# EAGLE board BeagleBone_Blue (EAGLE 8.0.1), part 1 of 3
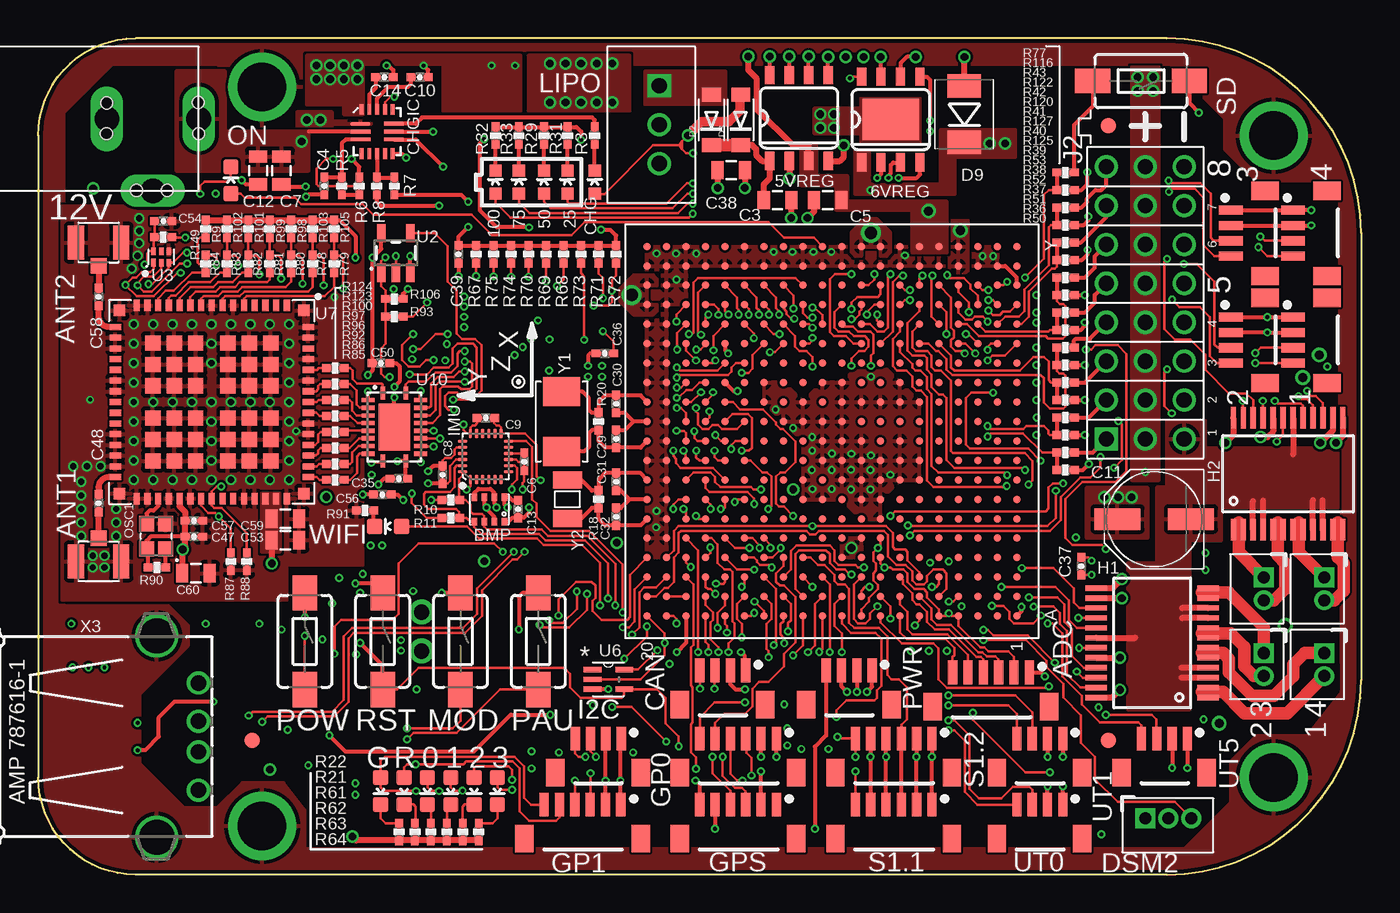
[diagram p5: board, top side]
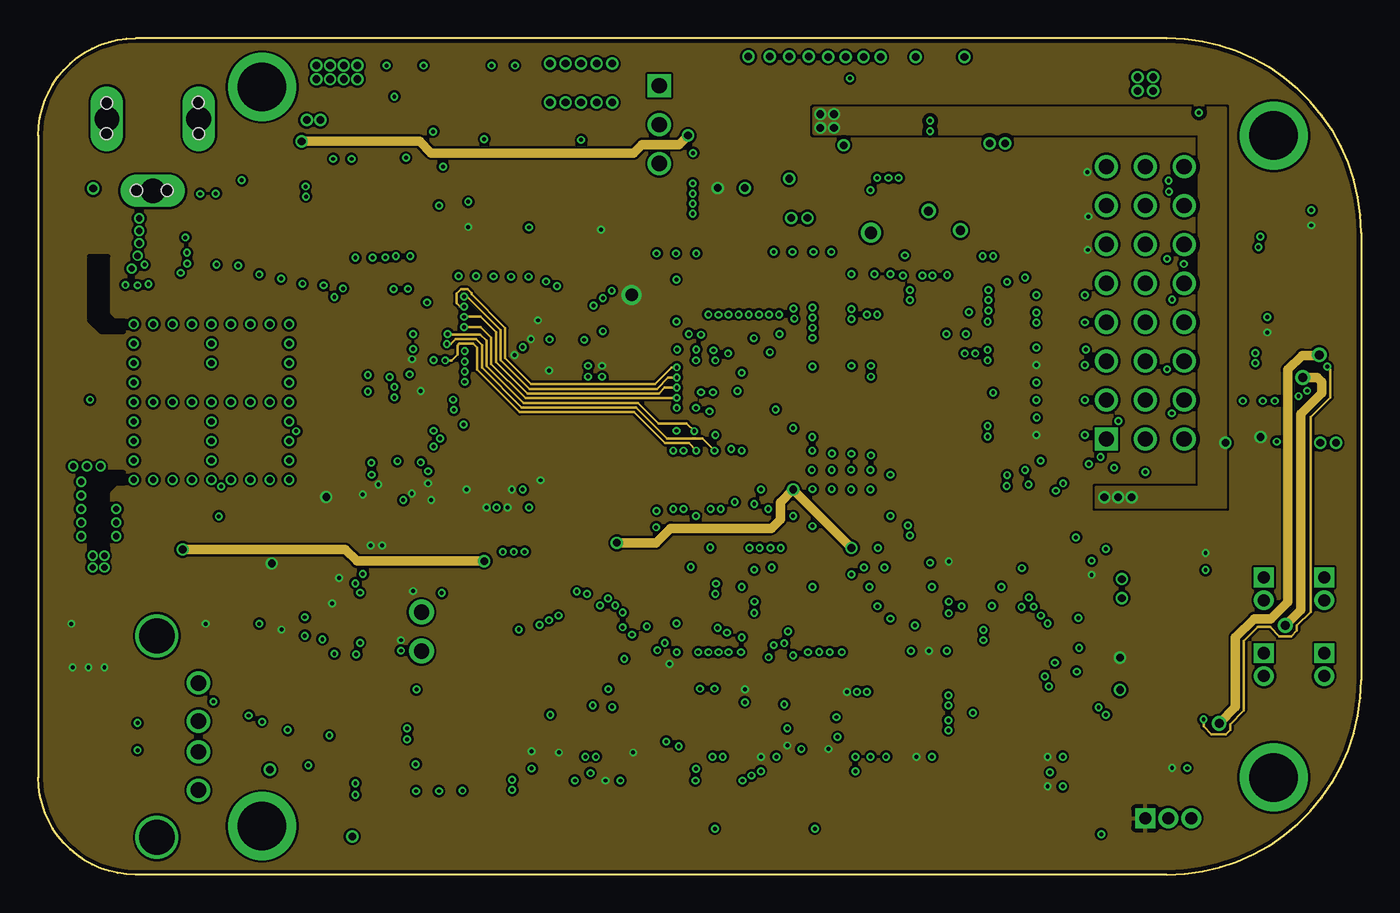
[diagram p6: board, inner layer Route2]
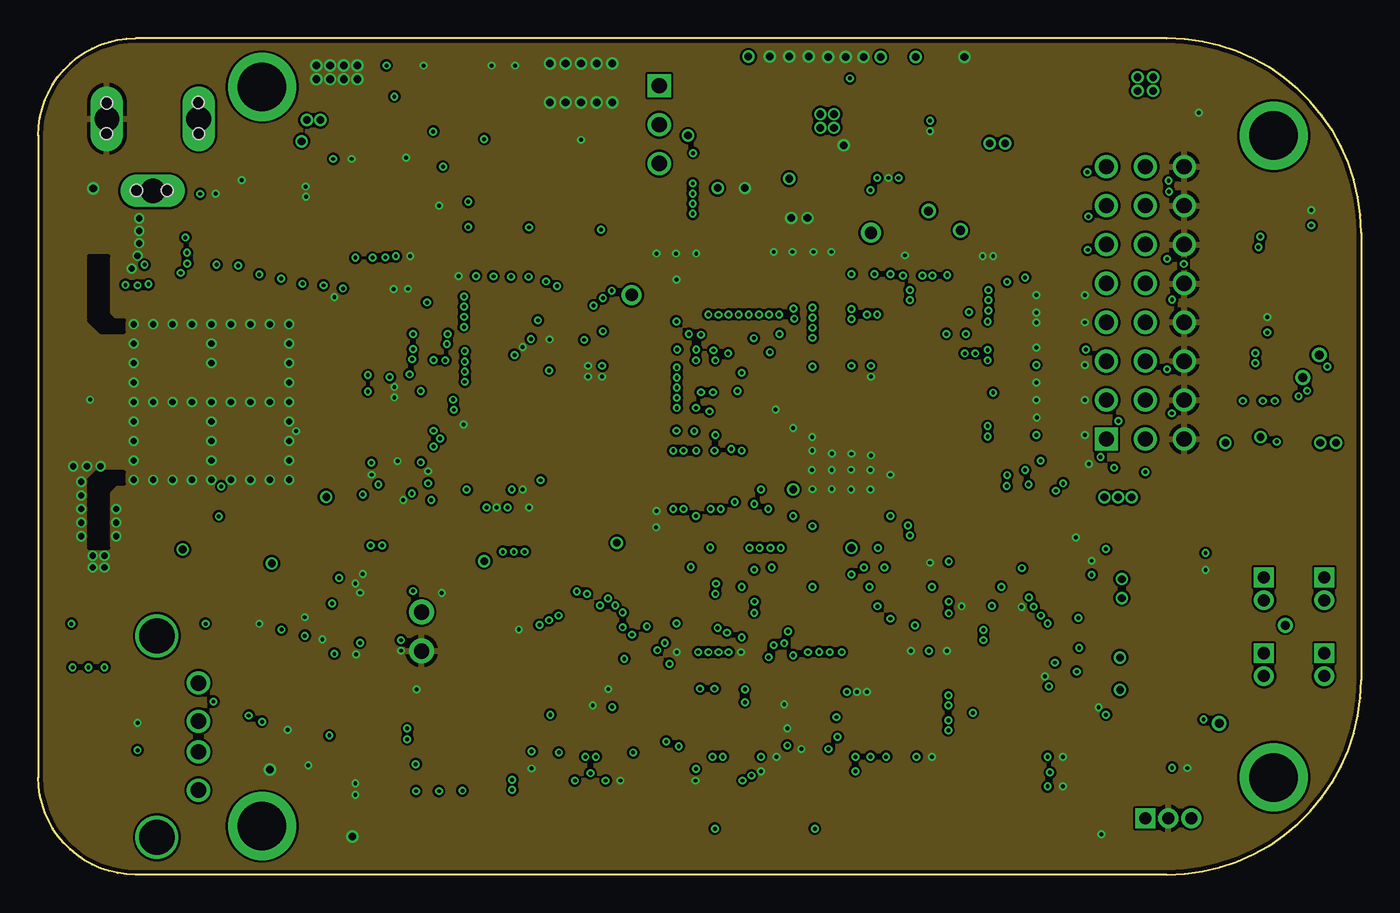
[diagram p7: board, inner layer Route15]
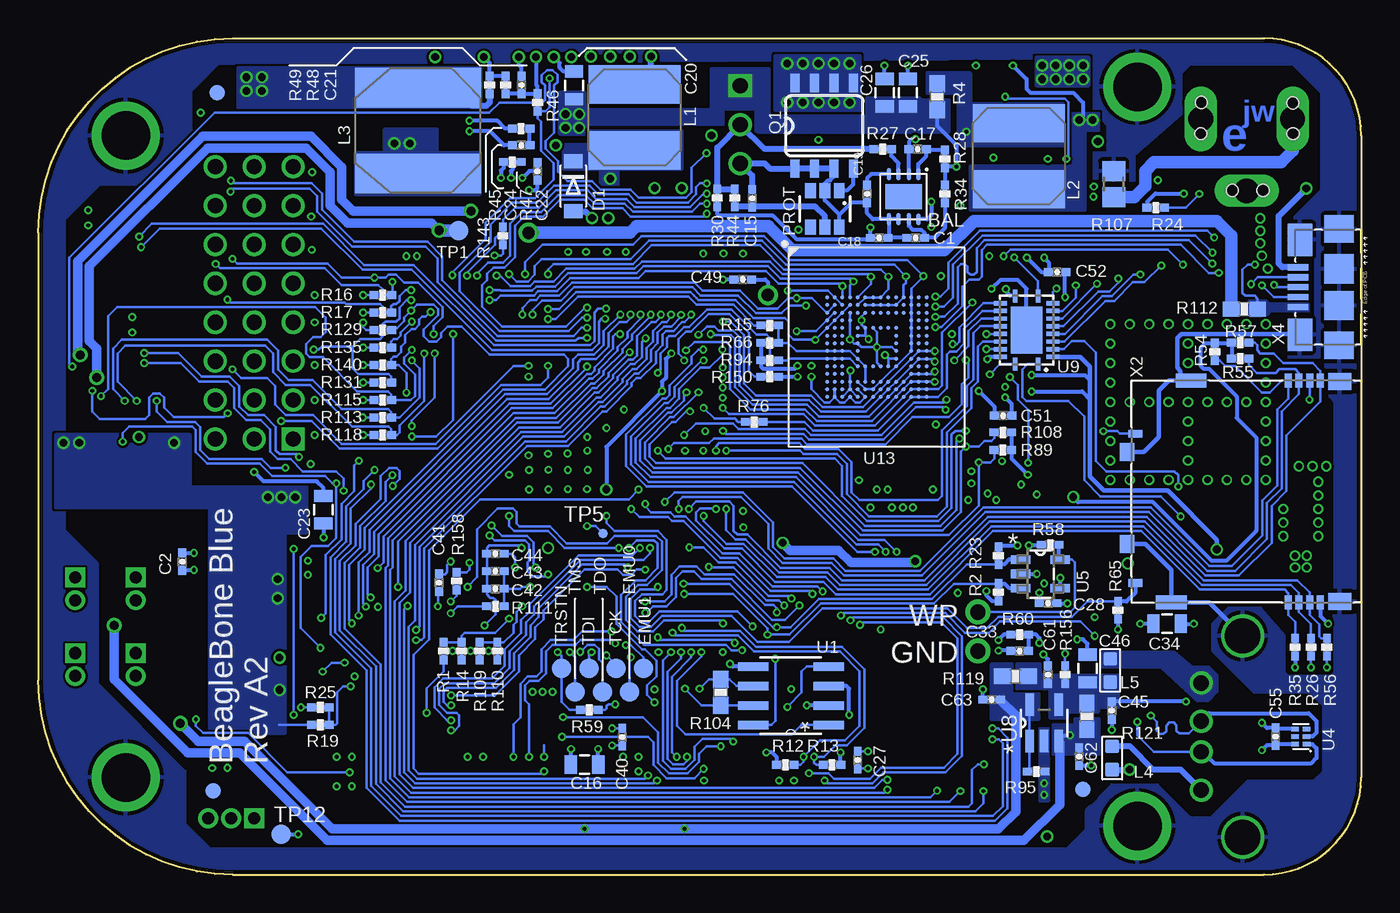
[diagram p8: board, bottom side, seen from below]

Size 86.36 x 54.61 mm. Coordinates in mm from the lower left corner, seen from the top.
Copper layers (1+2*15+16): Top 0.0178mm / dielectric 12mil / Route2 0.0356mm / dielectric 28mil / Route15 0.0356mm / dielectric 12mil / Bottom 0.0178mm
Design rules "SSC-EAGLE-4Lyr_v1.0.0.3 *": minimum track width 6mil, minimum drill 10mil, track to track 6mil, track to pad 6mil, pad to pad 6mil, via to via 6mil, smd to smd 6mil, copper to edge 10mil, drill to drill 8mil, minimum pad ring 10mil, minimum via ring 5mil, stop-mask expansion 3mil, vias tented up to drill 40mil, thermal gap 10mil
Net classes: 0 default: width 0.152 mm, drill 0.254 mm, clearance 0.152 mm; 1 ground: width 0.152 mm, drill 0.254 mm, clearance 0.152 mm; 2 usb: width 0.152 mm, drill 0.254 mm, clearance 0.152 mm; 3 power: width 0.152 mm, drill 0.254 mm, clearance 0.152 mm

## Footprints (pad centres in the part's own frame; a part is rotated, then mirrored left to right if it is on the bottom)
BEAGLEBONE_BLUE_LED-0603 = smd 1 x 1: A 0,-0.877; C 0,0.877
BEAGLEBONE_BLUE_SO08-TIGHT = smd 0.6 x 1.2: 1 -1.905,-2.8; 2 -0.635,-2.8; 3 0.635,-2.8; 4 1.905,-2.8; 5 1.905,2.8; 6 0.635,2.8; 7 -0.635,2.8; 8 -1.905,2.8
SO08-EXPOSED = smd 0.6 x 1.2: 1 -1.905,-2.8; 2 -0.635,-2.8; 3 0.635,-2.8; 4 1.905,-2.8; 5 1.905,2.8; 6 0.635,2.8; 7 -0.635,2.8; 8 -1.905,2.8 | smd 3.683 x 2.718: 9 0,0
PJ-102B_POWER_CON = drill 1.6 long: IN -6,0; OUT 0,0; OUT_CON -3,4.7 | hole 0.762: 0,-1.041; 0.025,0.965; -5.994,0.965; -5.969,-1.067; -1.93,4.674; -3.937,4.674
JST_SH_6 = smd 0.6 x 1.55: 1 5,0; 2 4,0; 3 3,0; 4 2,0; 5 1,0; 6 0,0 | smd 1.2 x 1.8: P$1 -1.3,-2.225; P$2 6.3,-2.225
U.FL-R-SMT-1 = smd 1.05 x 2.2: GND1 -1.475,0; GND2 1.475,0 | smd 1.05 x 1: SIG 0,-1.525
LED-0603 = smd 0.8 x 0.8: A 0,-0.75; C 0,0.75
8-SON_3X3MM = smd 0.305 x 0.813: 1 -0.965,-1.473; 2 -0.33,-1.473; 3 0.33,-1.473; 4 0.965,-1.473; 5 0.965,1.473; 6 0.33,1.473; 7 -0.33,1.473 | smd 0.305 x 0.787: 8 -0.965,1.473 | smd 2.4 x 1.651: PAD 0,0
BMP280 = smd 0.5 x 0.35: 1 0.8,0.975; 2 0.8,0.325; 3 0.8,-0.325; 4 0.8,-0.975; 5 -0.8,-0.975; 6 -0.8,-0.325; 7 -0.8,0.325; 8 -0.8,0.975
0402-CAP = smd 0.61 x 0.508: 1 -0.559,0; 2 0.559,0
0805 = smd 0.8 x 1.2: 1 -0.9,0; 2 0.9,0
PANASONIC_D = smd 3 x 1.4: + 2.4,0; - -2.4,0
JST_SH_4_SMD = smd 0.6 x 1.55: 1 0.46,1.27; 2 -0.54,1.27; 3 -1.54,1.27; 4 -2.54,1.27 | smd 1.2 x 1.8: P$1 -3.84,-0.955; P$2 1.728,-0.955
MP2615 = smd 1.295 x 0.254: 1 -1.092,0.508; 2 -1.092,0; 3 -1.092,-0.508; 9 1.092,-0.508; 10 1.092,0; 11 1.092,0.508 | smd 0.254 x 0.711: 4 -1.016,-1.448; 5 -0.508,-1.448; 6 0,-1.448; 7 0.508,-1.448; 8 1.016,-1.448; 12 1.016,1.448; 13 0.508,1.448; 14 0,1.448; 15 -0.508,1.448; 16 -1.016,1.448
ADAFRUIT_SOD-123FL = smd 0.91 x 1.22: A 1.637,0; C -1.637,0
DO-214AA = smd 1.524 x 2.184: A 1.841,0; C -1.841,0
JST_ZH_3 = drill 0.787 square: P$1 0,0 | drill 0.787: P$2 1.499,0; P$3 2.997,0
B1,27 = smd 1.27 x 1.27: TP 0,0
FIDUCIAL_40MIL = smd 1.016 x 1.016: P$1 0,0
GHI2_TESTPAD/W_HOLE_1X1 = drill 1 pad 1.626: P$1 0,0
SSOP24 = smd 0.348 x 1.397: 1 -3.575,-3.656; 2 -2.925,-3.656; 3 -2.275,-3.656; 4 -1.625,-3.656; 5 -0.975,-3.656; 6 -0.325,-3.656; 7 0.325,-3.656; 8 0.975,-3.656; 9 1.625,-3.656; 10 2.275,-3.656; 11 2.925,-3.656; 12 3.575,-3.656; 13 3.575,3.656; 14 2.925,3.656; 15 2.275,3.656; 16 1.625,3.656; 17 0.975,3.656; 18 0.325,3.656; 19 -0.325,3.656; 20 -0.975,3.656; 21 -1.625,3.656; 22 -2.275,3.656; 23 -2.925,3.656; 24 -3.575,3.656
QFN24G-0.4-3X3MM = smd 0.6 x 0.2: 1 -1.5,1; 2 -1.5,0.6; 3 -1.5,0.2; 4 -1.5,-0.2; 5 -1.5,-0.6; 6 -1.5,-1; 13 1.5,-1; 14 1.5,-0.6; 15 1.5,-0.2; 16 1.5,0.2; 17 1.5,0.6; 18 1.5,1 | smd 0.2 x 0.6: 7 -1,-1.5; 8 -0.6,-1.5; 9 -0.2,-1.5; 10 0.2,-1.5; 11 0.6,-1.5; 12 1,-1.5; 19 1,1.5; 20 0.6,1.5; 21 0.2,1.5; 22 -0.2,1.5; 23 -0.6,1.5; 24 -1,1.5
STRAWSON_EAGLE_LIB_3X8_0.1"_HEADER = drill 1 square: P$1 -2.54,-17.78 | drill 1: P$2 -2.54,-15.24; P$3 -2.54,-12.7; P$4 -2.54,-10.16; P$5 -2.54,-7.62; P$6 -2.54,-5.08; P$7 0,-17.78; P$8 0,-15.24; P$9 0,-12.7; P$10 0,-10.16; P$11 0,-7.62; P$12 0,-5.08; P$13 2.54,-17.78; P$14 2.54,-15.24; P$15 2.54,-12.7; P$16 2.54,-10.16; P$17 2.54,-7.62; P$18 2.54,-5.08; P$19 -2.54,-2.54; P$20 -2.54,0; P$21 0,-2.54; P$22 0,0; P$23 2.54,-2.54; P$24 2.54,0
SRN6045 = smd 2.5 x 6: 1 -2.175,-0.175; 2 2.125,-0.175
8X8MM_INDUCTOR = smd 2.591 x 8.204: 1 -2.794,0; 2 2.794,0
L0603 = smd 0.889 x 0.889: 1 -0.762,0; 2 0.762,0
JST_XH_3-PIN = drill 1 square: P$1 0,0 | drill 1: P$2 0,-2.54; P$3 0,-5.08
JST_ZH_2 = drill 0.787 pad 1.219 square: P$1 -0.749,0 | drill 0.787 pad 1.219: P$2 0.749,0
MOUNTING_HOLE = drill 3.175 pad 4.445: P$1 0,0
TACTILE-SWITCH-1101NE = smd 2.3 x 1.6: 1 -3.15,0; 2 3.15,0
NZ2520S = smd 1 x 1: 1 -0.825,-0.625; 2 0.825,-0.625; 3 0.825,0.625; 4 -0.825,0.625
SOT-236 = smd 0.991 x 0.711: 1 -1.194,0.94; 2 -1.194,0; 3 -1.194,-0.94; 4 1.194,-0.94; 5 1.194,0; 6 1.194,0.94
SO08-TIGHT = smd 0.6 x 1.2: 1 -1.905,-2.8; 2 -0.635,-2.8; 3 0.635,-2.8; 4 1.905,-2.8; 5 1.905,2.8; 6 0.635,2.8; 7 -0.635,2.8; 8 -1.905,2.8
0402-RES = smd 0.61 x 0.508: 1 -0.559,0; 2 0.559,0
0603-RES = smd 1.1 x 1: 1 -0.85,0; 2 0.85,0
R0805 = smd 1.3 x 1.5: 1 -0.85,0; 2 0.85,0
BEAGLEBONE_BLUE_OSD3358 = smd 0.5 x 0.5: A1 -12.065,-12.065; A2 -12.065,-10.795; A3 -12.065,-9.525; A4 -12.065,-8.255; A5 -12.065,-6.985; A6 -12.065,-5.715; A7 -12.065,-4.445; A8 -12.065,-3.175; A9 -12.065,-1.905; A10 -12.065,-0.635; A11 -12.065,0.635; A12 -12.065,1.905; A13 -12.065,3.175; A14 -12.065,4.445; A15 -12.065,5.715; A16 -12.065,6.985; A17 -12.065,8.255; A18 -12.065,9.525; A19 -12.065,10.795; A20 -12.065,12.065; B1 -10.795,-12.065; B2 -10.795,-10.795; B3 -10.795,-9.525; B4 -10.795,-8.255; B5 -10.795,-6.985; B6 -10.795,-5.715; B7 -10.795,-4.445; B8 -10.795,-3.175; B9 -10.795,-1.905; B10 -10.795,-0.635; B11 -10.795,0.635; B12 -10.795,1.905; B13 -10.795,3.175; B14 -10.795,4.445; B15 -10.795,5.715; B16 -10.795,6.985; B17 -10.795,8.255; B18 -10.795,9.525; B19 -10.795,10.795; B20 -10.795,12.065; C1 -9.525,-12.065; C2 -9.525,-10.795; C3 -9.525,-9.525; C4 -9.525,-8.255; C5 -9.525,-6.985; C6 -9.525,-5.715; C7 -9.525,-4.445; C8 -9.525,-3.175; C9 -9.525,-1.905; C10 -9.525,-0.635; C11 -9.525,0.635; C12 -9.525,1.905; C13 -9.525,3.175; C14 -9.525,4.445; C15 -9.525,5.715; C16 -9.525,6.985; C17 -9.525,8.255; C18 -9.525,9.525; C19 -9.525,10.795; C20 -9.525,12.065; D1 -8.255,-12.065; D2 -8.255,-10.795; D3 -8.255,-9.525; D4 -8.255,-8.255; D5 -8.255,-6.985; D6 -8.255,-5.715; D7 -8.255,-4.445; D8 -8.255,-3.175; D9 -8.255,-1.905; D10 -8.255,-0.635; D11 -8.255,0.635; D12 -8.255,1.905; D13 -8.255,3.175; D14 -8.255,4.445; D15 -8.255,5.715; D16 -8.255,6.985; D17 -8.255,8.255; D18 -8.255,9.525; D19 -8.255,10.795; D20 -8.255,12.065; E1 -6.985,-12.065; E2 -6.985,-10.795; E3 -6.985,-9.525; E4 -6.985,-8.255; E5 -6.985,-6.985; E6 -6.985,-5.715; E7 -6.985,-4.445; E8 -6.985,-3.175; E9 -6.985,-1.905; E10 -6.985,-0.635; E11 -6.985,0.635; E12 -6.985,1.905; E13 -6.985,3.175; E14 -6.985,4.445; E15 -6.985,5.715; E16 -6.985,6.985; E17 -6.985,8.255; E18 -6.985,9.525; E19 -6.985,10.795; E20 -6.985,12.065; F1 -5.715,-12.065; F2 -5.715,-10.795; F3 -5.715,-9.525; F4 -5.715,-8.255; F5 -5.715,-6.985; F6 -5.715,-5.715; F7 -5.715,-4.445; F8 -5.715,-3.175; F9 -5.715,-1.905; F10 -5.715,-0.635; F11 -5.715,0.635; F12 -5.715,1.905; F13 -5.715,3.175; F14 -5.715,4.445; F15 -5.715,5.715; F16 -5.715,6.985; F17 -5.715,8.255; F18 -5.715,9.525; F19 -5.715,10.795; F20 -5.715,12.065; G1 -4.445,-12.065; G2 -4.445,-10.795; G3 -4.445,-9.525; G4 -4.445,-8.255; G5 -4.445,-6.985; G6 -4.445,-5.715; G7 -4.445,-4.445; G8 -4.445,-3.175; G9 -4.445,-1.905; G10 -4.445,-0.635; G11 -4.445,0.635; G12 -4.445,1.905; G13 -4.445,3.175; G14 -4.445,4.445; G15 -4.445,5.715; G16 -4.445,6.985; G17 -4.445,8.255; G18 -4.445,9.525; G19 -4.445,10.795; G20 -4.445,12.065; H1 -3.175,-12.065; H2 -3.175,-10.795; H3 -3.175,-9.525; H4 -3.175,-8.255; H5 -3.175,-6.985; H6 -3.175,-5.715; H7 -3.175,-4.445; H8 -3.175,-3.175; H9 -3.175,-1.905; H10 -3.175,-0.635; H11 -3.175,0.635; H12 -3.175,1.905; H13 -3.175,3.175; H14 -3.175,4.445; H15 -3.175,5.715; H16 -3.175,6.985; H17 -3.175,8.255; H18 -3.175,9.525; H19 -3.175,10.795; H20 -3.175,12.065; J1 -1.905,-12.065; J2 -1.905,-10.795; J3 -1.905,-9.525; J4 -1.905,-8.255; J5 -1.905,-6.985; J6 -1.905,-5.715; J7 -1.905,-4.445; J8 -1.905,-3.175; J9 -1.905,-1.905; J10 -1.905,-0.635; J11 -1.905,0.635; J12 -1.905,1.905; J13 -1.905,3.175; J14 -1.905,4.445; J15 -1.905,5.715; J16 -1.905,6.985; J17 -1.905,8.255; J18 -1.905,9.525; J19 -1.905,10.795; J20 -1.905,12.065; K1 -0.635,-12.065; K2 -0.635,-10.795; K3 -0.635,-9.525; K4 -0.635,-8.255; K5 -0.635,-6.985; K6 -0.635,-5.715; K7 -0.635,-4.445; K8 -0.635,-3.175; K9 -0.635,-1.905; K10 -0.635,-0.635; K11 -0.635,0.635; K12 -0.635,1.905; K13 -0.635,3.175; K14 -0.635,4.445; K15 -0.635,5.715; K16 -0.635,6.985; K17 -0.635,8.255; K18 -0.635,9.525; K19 -0.635,10.795; K20 -0.635,12.065; L1 0.635,-12.065; L2 0.635,-10.795; L3 0.635,-9.525; L4 0.635,-8.255; L5 0.635,-6.985; L6 0.635,-5.715; L7 0.635,-4.445; L8 0.635,-3.175; L9 0.635,-1.905; L10 0.635,-0.635; L11 0.635,0.635; L12 0.635,1.905; L13 0.635,3.175; L14 0.635,4.445; L15 0.635,5.715; L16 0.635,6.985; L17 0.635,8.255; L18 0.635,9.525; L19 0.635,10.795; L20 0.635,12.065; M1 1.905,-12.065; M2 1.905,-10.795; M3 1.905,-9.525; M4 1.905,-8.255; M5 1.905,-6.985; M6 1.905,-5.715; M7 1.905,-4.445; M8 1.905,-3.175; M9 1.905,-1.905; M10 1.905,-0.635; M11 1.905,0.635; M12 1.905,1.905; M13 1.905,3.175; M14 1.905,4.445; M15 1.905,5.715; M16 1.905,6.985; M17 1.905,8.255; M18 1.905,9.525; M19 1.905,10.795; M20 1.905,12.065; N1 3.175,-12.065; N2 3.175,-10.795; N3 3.175,-9.525; N4 3.175,-8.255; N5 3.175,-6.985; N6 3.175,-5.715; N7 3.175,-4.445; N8 3.175,-3.175; N9 3.175,-1.905; N10 3.175,-0.635; N11 3.175,0.635; N12 3.175,1.905; N13 3.175,3.175; N14 3.175,4.445; N15 3.175,5.715; N16 3.175,6.985; N17 3.175,8.255; N18 3.175,9.525; N19 3.175,10.795; N20 3.175,12.065; P1 4.445,-12.065; P2 4.445,-10.795; P3 4.445,-9.525; P4 4.445,-8.255; P5 4.445,-6.985; P6 4.445,-5.715; P7 4.445,-4.445; P8 4.445,-3.175; P9 4.445,-1.905; P10 4.445,-0.635; P11 4.445,0.635; P12 4.445,1.905; P13 4.445,3.175; P14 4.445,4.445; P15 4.445,5.715; P16 4.445,6.985; P17 4.445,8.255; P18 4.445,9.525; P19 4.445,10.795; P20 4.445,12.065; R1 5.715,-12.065; R2 5.715,-10.795; R3 5.715,-9.525; R4 5.715,-8.255; R5 5.715,-6.985; R6 5.715,-5.715; R7 5.715,-4.445; R8 5.715,-3.175; R9 5.715,-1.905; R10 5.715,-0.635; R11 5.715,0.635; R12 5.715,1.905; R13 5.715,3.175; R14 5.715,4.445; R15 5.715,5.715; R16 5.715,6.985; R17 5.715,8.255; R18 5.715,9.525; R19 5.715,10.795; R20 5.715,12.065; T1 6.985,-12.065; T2 6.985,-10.795; T3 6.985,-9.525; T4 6.985,-8.255; T5 6.985,-6.985; T6 6.985,-5.715; T7 6.985,-4.445; T8 6.985,-3.175; T9 6.985,-1.905; T10 6.985,-0.635; T11 6.985,0.635; T12 6.985,1.905; T13 6.985,3.175; T14 6.985,4.445; T15 6.985,5.715; T16 6.985,6.985; T17 6.985,8.255; T18 6.985,9.525; T19 6.985,10.795; T20 6.985,12.065; U1 8.255,-12.065; U2 8.255,-10.795; U3 8.255,-9.525; U4 8.255,-8.255; U5 8.255,-6.985; U6 8.255,-5.715; U7 8.255,-4.445; U8 8.255,-3.175; U9 8.255,-1.905; U10 8.255,-0.635; U11 8.255,0.635; U12 8.255,1.905; U13 8.255,3.175; U14 8.255,4.445; U15 8.255,5.715; U16 8.255,6.985; U17 8.255,8.255; U18 8.255,9.525; U19 8.255,10.795; U20 8.255,12.065; V1 9.525,-12.065; V2 9.525,-10.795; V3 9.525,-9.525; V4 9.525,-8.255; V5 9.525,-6.985; V6 9.525,-5.715; V7 9.525,-4.445; V8 9.525,-3.175; V9 9.525,-1.905; V10 9.525,-0.635; V11 9.525,0.635; V12 9.525,1.905; V13 9.525,3.175; V14 9.525,4.445; V15 9.525,5.715; V16 9.525,6.985; V17 9.525,8.255; V18 9.525,9.525; V19 9.525,10.795; V20 9.525,12.065; W1 10.795,-12.065; W2 10.795,-10.795; W3 10.795,-9.525; W4 10.795,-8.255; W5 10.795,-6.985; W6 10.795,-5.715; W7 10.795,-4.445; W8 10.795,-3.175; W9 10.795,-1.905; W10 10.795,-0.635; W11 10.795,0.635; W12 10.795,1.905; W13 10.795,3.175; W14 10.795,4.445; W15 10.795,5.715; W16 10.795,6.985; W17 10.795,8.255; W18 10.795,9.525; W19 10.795,10.795; W20 10.795,12.065; Y1 12.065,-12.065; Y2 12.065,-10.795; Y3 12.065,-9.525; Y4 12.065,-8.255; Y5 12.065,-6.985; Y6 12.065,-5.715; Y7 12.065,-4.445; Y8 12.065,-3.175; Y9 12.065,-1.905; Y10 12.065,-0.635; Y11 12.065,0.635; Y12 12.065,1.905; Y13 12.065,3.175; Y14 12.065,4.445; Y15 12.065,5.715; Y16 12.065,6.985; Y17 12.065,8.255; Y18 12.065,9.525; Y19 12.065,10.795; Y20 12.065,12.065
BEAGLEBONE_BLUE_B0,65 = smd 0.635 x 0.635: TP 0,0
BEAGLEBONE_BLUE_D8 = smd 1.981 x 0.559: 1 -2.464,1.905; 2 -2.464,0.635; 3 -2.464,-0.635; 4 -2.464,-1.905; 5 2.464,-1.905; 6 2.464,-0.635; 7 2.464,0.635; 8 2.464,1.905
BEAGLEBONE_BLUE_SOT23-5 = smd 0.55 x 1.2: 1 -0.95,-1.3; 2 0,-1.3; 3 0.95,-1.3; 4 0.95,1.3; 5 -0.95,1.3
SON-6(TI)-DRY = smd 0.3 x 0.52: 1 -0.5,-0.38 | smd 0.3 x 0.49: 2 0,-0.375; 3 0.5,-0.375; 4 0.5,0.375; 5 0,0.375; 6 -0.5,0.375
SOT95P290X145-5N = smd 1.27 x 0.559: 1 -1.295,0.94; 2 -1.295,0; 3 -1.295,-0.94; 4 1.295,-0.94; 5 1.295,0.94
BEAGLEBONE_BLUE_DCK5 = smd 1.168 x 0.356: 1 -1.041,0.65; 2 -1.041,0; 3 -1.041,-0.65; 4 1.041,-0.65; 5 1.041,0.65
MOC-100(TI) = smd 0.75 x 0.75: 1 -6.025,-5.975; 17 6.025,-5.975; 33 6.025,5.975; 49 -6.025,5.975 | smd 0.4 x 0.75: 2 -4.9,-6.3; 3 -4.2,-6.3; 4 -3.5,-6.3; 5 -2.8,-6.3; 6 -2.1,-6.3; 7 -1.4,-6.3; 8 -0.7,-6.3; 9 0,-6.3; 10 0.7,-6.3; 11 1.4,-6.3; 12 2.1,-6.3; 13 2.8,-6.3; 14 3.5,-6.3; 15 4.2,-6.3; 16 4.9,-6.3; 34 4.9,6.3; 35 4.2,6.3; 36 3.5,6.3; 37 2.8,6.3; 38 2.1,6.3; 39 1.4,6.3; 40 0.7,6.3; 41 0,6.3; 42 -0.7,6.3; 43 -1.4,6.3; 44 -2.1,6.3; 45 -2.8,6.3; 46 -3.5,6.3; 47 -4.2,6.3; 48 -4.9,6.3 | smd 0.75 x 0.4: 18 6.3,-4.9; 19 6.3,-4.2; 20 6.3,-3.5; 21 6.3,-2.8; 22 6.3,-2.1; 23 6.3,-1.4; 24 6.3,-0.7; 25 6.3,0; 26 6.3,0.7; 27 6.3,1.4; 28 6.3,2.1; 29 6.3,2.8; 30 6.3,3.5; 31 6.3,4.2; 32 6.3,4.9; 50 -6.3,4.9; 51 -6.3,4.2; 52 -6.3,3.5; 53 -6.3,2.8; 54 -6.3,2.1; 55 -6.3,1.4; 56 -6.3,0.7; 57 -6.3,0; 58 -6.3,-0.7; 59 -6.3,-1.4; 60 -6.3,-2.1; 61 -6.3,-2.8; 62 -6.3,-3.5; 63 -6.3,-4.2; 64 -6.3,-4.9 | smd 1 x 1: G1 -3.85,-3.85; G2 -2.45,-3.85; G3 -1.05,-3.85; G4 1.05,-3.85; G5 2.45,-3.85; G6 3.85,-3.85; G7 -3.85,-2.45; G8 -2.45,-2.45; G9 -1.05,-2.45; G10 1.05,-2.45; G11 2.45,-2.45; G12 3.85,-2.45; G13 -3.85,-1.05; G14 -2.45,-1.05; G15 -1.05,-1.05; G16 1.05,-1.05; G17 2.45,-1.05; G18 3.85,-1.05; G19 -3.85,1.05; G20 -2.45,1.05; G21 -1.05,1.05; G22 1.05,1.05; G23 2.45,1.05; G24 3.85,1.05; G25 -3.85,2.45; G26 -2.45,2.45; G27 -1.05,2.45; G28 1.05,2.45; G29 2.45,2.45; G30 3.85,2.45; G31 -3.85,3.85; G32 -2.45,3.85; G33 -1.05,3.85; G34 1.05,3.85; G35 2.45,3.85; G36 3.85,3.85
DBV5 = smd 1.473 x 0.559: 1 -1.194,0.95; 2 -1.194,0; 3 -1.194,-0.95; 4 1.194,-0.95; 5 1.194,0.95
R-PVQFN-N20(TI) = smd 0.85 x 0.28: 1 -2.225,-0.75; 10 2.225,-0.75; 11 2.225,0.75; 20 -2.225,0.75 | smd 0.28 x 0.85: 2 -1.75,-1.725; 3 -1.25,-1.725; 4 -0.75,-1.725; 5 -0.25,-1.725; 6 0.25,-1.725; 7 0.75,-1.725; 8 1.25,-1.725; 9 1.75,-1.725; 12 1.75,1.725; 13 1.25,1.725; 14 0.75,1.725; 15 0.25,1.725; 16 -0.25,1.725; 17 -0.75,1.725; 18 -1.25,1.725; 19 -1.75,1.725 | smd 3.05 x 2.05: TP 0,0
MICRON_EMMC_153 = smd 0.245 x 0.245: A1 -3.25,3.25; A2 -2.75,3.25; A3 -2.25,3.25; A4 -1.75,3.25; A5 -1.25,3.25; A6 -0.75,3.25; A7 -0.25,3.25; A8 0.25,3.25; A9 0.75,3.25; A10 1.25,3.25; A11 1.75,3.25; A12 2.25,3.25; A13 2.75,3.25; A14 3.25,3.25; B1 -3.25,2.75; B2 -2.75,2.75; B3 -2.25,2.75; B4 -1.75,2.75; B5 -1.25,2.75; B6 -0.75,2.75; B7 -0.25,2.75; B8 0.25,2.75; B9 0.75,2.75; B10 1.25,2.75; B11 1.75,2.75; B12 2.25,2.75; B13 2.75,2.75; B14 3.25,2.75; C1 -3.25,2.25; C2 -2.75,2.25; C3 -2.25,2.25; C4 -1.75,2.25; C5 -1.25,2.25; C6 -0.75,2.25; C7 -0.25,2.25; C8 0.25,2.25; C9 0.75,2.25; C10 1.25,2.25; C11 1.75,2.25; C12 2.25,2.25; C13 2.75,2.25; C14 3.25,2.25; D1 -3.25,1.75; D2 -2.75,1.75; D3 -2.25,1.75; D4 -1.75,1.75; D12 2.25,1.75; D13 2.75,1.75; D14 3.25,1.75; E1 -3.25,1.25; E2 -2.75,1.25; E3 -2.25,1.25; E5 -1.25,1.25; E6 -0.75,1.25; E7 -0.25,1.25; E8 0.25,1.25; E9 0.75,1.25; E10 1.25,1.25; E12 2.25,1.25; E13 2.75,1.25; E14 3.25,1.25; F1 -3.25,0.75; F2 -2.75,0.75; F3 -2.25,0.75; F5 -1.25,0.75; F10 1.25,0.75; F12 2.25,0.75; F13 2.75,0.75; F14 3.25,0.75; G1 -3.25,0.25; G2 -2.75,0.25; G3 -2.25,0.25; G5 -1.25,0.25; G10 1.25,0.25; G12 2.25,0.25; G13 2.75,0.25; G14 3.25,0.25; H1 -3.25,-0.25; H2 -2.75,-0.25; H3 -2.25,-0.25; H5 -1.25,-0.25; H10 1.25,-0.25; H12 2.25,-0.25; H13 2.75,-0.25; H14 3.25,-0.25; J1 -3.25,-0.75; J2 -2.75,-0.75; J3 -2.25,-0.75; J5 -1.25,-0.75; J10 1.25,-0.75; J12 2.25,-0.75; J13 2.75,-0.75; J14 3.25,-0.75; K1 -3.25,-1.25; K2 -2.75,-1.25; K3 -2.25,-1.25; K5 -1.25,-1.25; K6 -0.75,-1.25; K7 -0.25,-1.25; K8 0.25,-1.25; K9 0.75,-1.25; K10 1.25,-1.25; K12 2.25,-1.25; K13 2.75,-1.25; K14 3.25,-1.25; L1 -3.25,-1.75; L2 -2.75,-1.75; L3 -2.25,-1.75; L12 2.25,-1.75; L13 2.75,-1.75; L14 3.25,-1.75; M1 -3.25,-2.25; M2 -2.75,-2.25; M3 -2.25,-2.25; M4 -1.75,-2.25; M5 -1.25,-2.25; M6 -0.75,-2.25; M7 -0.25,-2.25; M8 0.25,-2.25; M9 0.75,-2.25; M10 1.25,-2.25; M11 1.75,-2.25; M12 2.25,-2.25; M13 2.75,-2.25; M14 3.25,-2.25; N1 -3.25,-2.75; N2 -2.75,-2.75; N3 -2.25,-2.75; N4 -1.75,-2.75; N5 -1.25,-2.75; N6 -0.75,-2.75; N7 -0.25,-2.75; N8 0.25,-2.75; N9 0.75,-2.75; N10 1.25,-2.75; N11 1.75,-2.75; N12 2.25,-2.75; N13 2.75,-2.75; N14 3.25,-2.75; P1 -3.25,-3.25; P2 -2.75,-3.25; P3 -2.25,-3.25; P4 -1.75,-3.25; P5 -1.25,-3.25; P6 -0.75,-3.25; P7 -0.25,-3.25; P8 0.25,-3.25; P9 0.75,-3.25; P10 1.25,-3.25; P11 1.75,-3.25; P12 2.25,-3.25; P13 2.75,-3.25; P14 3.25,-3.25
SCHA5B0200 = smd 0.9 x 0.45: 1 -7.25,3.365; 2 -7.25,2.665; 3 -7.25,1.965; 4 -7.25,1.265; 5 7.25,1.265; 6 7.25,1.965; 7 7.25,2.665; 8 7.25,3.365 | smd 0.5 x 0.9: CD -5.975,13.35; GND 3.775,13.35 | smd 0.9 x 2: CGND1 -7.25,11; CGND4 7.25,9.7 | smd 1.1 x 1.5: CGND2 -7.188,0; CGND3 7.188,0 | smd 1.2 x 0.95: CGND5 2.575,13.9; CGND6 -3.425,13.9
USB_HOST_HORIZONTAL_W/CHASSIS_GND = drill 1: 1 -3.5,12.99; 2 -1,12.99; 3 1,12.99; 4 3.5,12.99 | drill 2.3: 5 -6.57,10.28; 6 6.57,10.28
10118192-0001LF(MICRO-USB-B-AMPHENOL-FCI) = smd 1.8 x 1.9: CGND1 -3.8,0; CGND4 3.8,0 | smd 1.9 x 1.9: CGND2 -1.2,0; CGND3 1.2,0 | smd 2.1 x 1.6: CGND5 3.1,2.55; CGND6 -3.1,2.55 | smd 0.4 x 1.35: D+ 0,2.675; D- -0.65,2.675; GND 1.3,2.675; ID 0.65,2.675; VBUS -1.3,2.675
CRYSTAL_5X3.2MM = smd 1.9 x 2.4: 1 -1.95,0; 2 1.95,0
CRYSTAL_3.2X1.5 = smd 1.1 x 1.9: P$1 -1.25,0; P$2 1.25,0

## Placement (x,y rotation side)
0  BLUE  [BEAGLEBONE_BLUE_LED-0603]  25.4,5.46 180 top
1  BLUE  [BEAGLEBONE_BLUE_LED-0603]  26.92,5.46 180 top
2  BLUE  [BEAGLEBONE_BLUE_LED-0603]  28.45,5.46 180 top
3  BLUE  [BEAGLEBONE_BLUE_LED-0603]  29.97,5.46 180 top
5VREG  AP1509SOIC-8-TIGHT  [BEAGLEBONE_BLUE_SO08-TIGHT]  49.66,49.4 0 top
6VREG  AOZ1284  [SO08-EXPOSED]  55.65,49.3 0 top
12V  PJ-102B_POWER_CON  [PJ-102B_POWER_CON]  4.47,49.35 180 top
ADC  JST_SH_6  [JST_SH_6]  59.69,13.21 0 top
ANT1  U.FL-R-SMT-1(10)  [U.FL-R-SMT-1]  3.94,20.45 180 top
ANT2  U.FL-R-SMT-1(10)  [U.FL-R-SMT-1]  3.94,41.27 0 top
B0  RED  [LED-0603]  34.54,45.21 0 top
B1  GREEN  [LED-0603]  33.02,45.21 0 top
B2  GREEN  [LED-0603]  31.37,45.21 0 top
B3  GREEN  [LED-0603]  29.84,45.21 0 top
BAL  BQ29209  [8-SON_3X3MM]  29.87,44.27 180 bottom
BMP  BMP280  [BMP280]  29.44,23.85 270 top
BOARD  [BEAGLEBONE_BLUE_NO_HOLES]  0,54.61 270 top
C1  0.1uF  [0402-CAP]  29.08,41.58 180 bottom
C2  0.1uF  [0402-CAP]  76.96,20.45 90 bottom
C3  10uF  [0805]  48.26,44.04 0 top
C4  1uF  [0402-CAP]  18.67,44.96 90 top
C5  10uF  [0805]  51.54,44.04 180 top
C6  0.1uF  [0402-CAP]  31.72,26.95 270 top
C7  10uF  [0805]  15.88,45.97 270 top
C8  0.1uF  [0402-CAP]  26.39,26.11 90 top
C9  0.1uF  [0402-CAP]  29.21,29.82 0 top
C10  1uF  [0402-CAP]  24.89,52.07 180 top
C11  100uF 16V  [PANASONIC_D]  72.85,23.22 180 top
C12  10uF  [0805]  14.35,45.97 270 top
C13  0.1uF  [0402-CAP]  31.32,23.88 270 top
C14  0.1uF  [0402-CAP]  22.61,52.07 0 top
C15  0.1uF  [0402-CAP]  39.75,44.17 270 bottom
C16  10uF  [0805]  50.7,7.19 0 bottom
C17  0.1uF  [0402-CAP]  28.96,47.37 0 bottom
C18  0.1uF  [0402-CAP]  31.47,41.58 180 bottom
C19  0.1uF  [0402-CAP]  32.26,44.45 270 bottom
C20  10uF  [0805]  51.38,51.54 270 bottom
C21  0.1uF  [0402-CAP]  54.81,51.56 90 bottom
C22  0.1uF  [0402-CAP]  53.77,45.92 270 bottom
C23  10uF  [0805]  67.74,23.83 90 bottom
C24  0.1uF  [0402-CAP]  54.84,47.62 0 bottom
C25  10uF  [0805]  29.59,51.05 90 bottom
C26  10uF  [0805]  31.11,51.05 90 bottom
C27  0.1uF  [0402-CAP]  32.87,7.49 270 bottom
C28  0.1uF  [0402-CAP]  20.45,17.73 180 bottom
C29  10pF  [0402-CAP]  37.72,28.45 90 top
C30  10pF  [0402-CAP]  37.72,30.73 270 top
C31  10pF  [0402-CAP]  37.72,25.65 270 top
C32  10pF  [0402-CAP]  37.72,23.37 270 top
C33  2.2uF  [0402-CAP]  22.3,14.6 180 bottom
C34  10uF  [0805]  12.67,16.38 0 bottom
C35  0.1uF  [0402-CAP]  23.55,25.86 180 top
C36  2.2uF  [0402-CAP]  36.98,34.04 180 top
C37  0.1uF  [0402-CAP]  68.08,20.15 90 top
C38  10uF  [0805]  45.24,46 0 top
C39  0.1uF  [0402-CAP]  27.43,40.51 270 top
C40  0.1uF  [0402-CAP]  48.23,8.99 90 bottom
C41  0.1uF  [0402-CAP]  60.2,19.05 270 bottom
C42  1nF  [0402-CAP]  56.52,18.67 180 bottom
C43  0.1uF  [0402-CAP]  56.52,19.81 180 bottom
C44  0.1uF  [0402-CAP]  56.52,20.95 180 bottom
C45  0.1uF  [0402-CAP]  16.28,10.72 270 bottom
C46  10uF  [0805]  17.87,13.46 90 bottom
C47  0.1uF  [0402-CAP]  10.16,22.07 0 top
C48  10pF  [0402-CAP]  3.94,24.26 90 top
C49  0.1uF  [0402-CAP]  40.36,38.86 0 bottom
C50  0.1uF  [0402-CAP]  22.38,33.4 0 top
C51  0.1uF  [0402-CAP]  23.37,29.97 180 bottom
C52  0.1uF  [0402-CAP]  19.84,39.34 0 bottom
C53  10uF  [0805]  16.13,23.24 0 top
C54  0.1uF  [0402-CAP]  8.15,42.67 0 top
C55  0.1uF  [0402-CAP]  5.59,9.02 90 bottom
C56  0.1uF  [0402-CAP]  22.45,24.82 0 top
C57  1uF  [0402-CAP]  10.16,23.11 180 top
C58  10pF  [0402-CAP]  3.94,37.72 270 top
C59  10uF  [0805]  16.13,21.84 0 top
C60  10uF  [0805]  10.29,19.69 180 top
C61  1uF  [0402-CAP]  20.45,13.06 270 bottom
C62  0.22uF  [0402-CAP]  18.41,7.7 270 bottom
C63  0.22uF  [0402-CAP]  24.13,11.43 180 bottom
CAN  JST_SH_4  [JST_SH_4_SMD]  45.72,12.06 0 top
CHG  GRN  [LED-0603]  36.32,45.21 0 top
CHGIC  MP2615  [MP2615]  22.12,48.51 0 top
D1  [ADAFRUIT_SOD-123FL]  51.44,44.96 270 bottom
D2  [ADAFRUIT_SOD-123FL]  43.94,49.28 90 top
D3  [ADAFRUIT_SOD-123FL]  45.85,49.28 90 top
D9  [DO-214AA]  60.45,49.66 90 top
DSM2  JST_ZH_3  [JST_ZH_3]  72.26,3.68 0 top
E1  JST_SH_4  [JST_SH_4_SMD]  83.19,35.94 90 top
E2  JST_SH_4  [JST_SH_4_SMD]  79.12,35.94 90 top
E3  JST_SH_4  [JST_SH_4_SMD]  79.12,42.93 90 top
E4  JST_SH_4  [JST_SH_4_SMD]  83.19,42.93 90 top
EMU0  TPSQB1,27  [B1,27]  47.75,11.94 0 bottom
EMU1  TPSQB1,27  [B1,27]  46.86,13.46 0 bottom
FUD1  FIDUCIAL  [FIDUCIAL_40MIL]  13.97,8.76 0 top
FUD2  FIDUCIAL  [FIDUCIAL_40MIL]  69.85,8.76 0 top
FUD3  FIDUCIAL  [FIDUCIAL_40MIL]  69.85,48.89 0 top
FUD4  FIDUCIAL  [FIDUCIAL_40MIL]  74.93,5.46 0 bottom
FUD5  FIDUCIAL  [FIDUCIAL_40MIL]  74.68,51.05 0 bottom
FUD6  FIDUCIAL  [FIDUCIAL_40MIL]  18.16,5.59 0 bottom
G  GREEN  [BEAGLEBONE_BLUE_LED-0603]  22.35,5.46 180 top
GND  GHI2_TESTPAD/W_HOLE_1X1  [GHI2_TESTPAD/W_HOLE_1X1]  25.02,14.6 0 bottom
GP0  JST_SH_6  [JST_SH_6]  43.18,8.89 0 top
GP1  JST_SH_6  [JST_SH_6]  33.02,4.57 0 top
GPS  JST_SH_6  [JST_SH_6]  43.18,4.57 0 top
H1  TB6612FNG  [SSOP24]  72.72,15.14 90 top
H2  TB6612FNG  [SSOP24]  81.58,26.17 0 top
I2C  JST_SH_4  [JST_SH_4_SMD]  37.59,7.62 0 top
IMU  MPU-9250  [QFN24G-0.4-3X3MM]  29.21,27.3 90 top
J2  STRAWSON_EAGLE_LIB_SERVO_HEADERS_8X  [STRAWSON_EAGLE_LIB_3X8_0.1"_HEADER]  72.26,46.23 0 top
L1  6.8uH  [SRN6045]  47.6,49.47 90 bottom
L2  6.8uH  [SRN6045]  22.53,46.94 90 bottom
L3  3.6 uH  [8X8MM_INDUCTOR]  61.57,48.59 90 bottom
L4  120  [L0603]  16.26,7.62 90 bottom
L5  120  [L0603]  16.38,13.34 90 bottom
LIPO  BATTERY  [JST_XH_3-PIN]  40.54,51.51 0 top
M1  JST_ZH_2  [JST_ZH_2]  83.95,13.72 270 top
M2  JST_ZH_2  [JST_ZH_2]  80.01,13.72 270 top
M3  JST_ZH_2  [JST_ZH_2]  80.01,18.67 270 top
M4  JST_ZH_2  [JST_ZH_2]  83.95,18.67 270 top
MGT1  MOUNTING_HOLE  [MOUNTING_HOLE]  14.61,51.44 0 top
MGT2  MOUNTING_HOLE  [MOUNTING_HOLE]  80.64,48.26 0 top
MGT3  MOUNTING_HOLE  [MOUNTING_HOLE]  80.64,6.35 0 top
MGT4  MOUNTING_HOLE  [MOUNTING_HOLE]  14.61,3.17 0 top
MOD  SWITCH-MOMENTARY-2SMD-1101NE  [TACTILE-SWITCH-1101NE]  27.56,15.24 270 top
ON  BLUE  [BEAGLEBONE_BLUE_LED-0603]  12.57,45.34 0 top
OSC1  NZ2520SB-32.768KHZ-NSA3534C  [NZ2520S]  7.7,22.1 90 top
PAU  SWITCH-MOMENTARY-2SMD-1101NE  [TACTILE-SWITCH-1101NE]  32.64,15.24 270 top
POW  SWITCH-MOMENTARY-2SMD-1101NE  [TACTILE-SWITCH-1101NE]  17.4,15.24 270 top
PROT  S-8261  [SOT-236]  35.01,43.47 270 bottom
PWR  JST_SH_4  [JST_SH_4_SMD]  53.98,12.06 0 top
Q1  MOSFET-N  [SO08-TIGHT]  35.05,48.89 0 bottom
R  RED  [BEAGLEBONE_BLUE_LED-0603]  23.88,5.46 180 top
R1  47k  [0402-RES]  59.89,14.6 90 bottom
R2  1.5K  [0402-RES]  23.67,18.44 270 bottom
R3  1k  [0402-RES]  36.32,48.26 270 top
R4  0.1  [0603-RES]  27.69,50.8 90 bottom
R5  10k  [0402-RES]  19.81,44.96 90 top
R6  10k  [0402-RES]  20.95,44.96 270 top
R7  4.7k  [0402-RES]  23.24,44.96 90 top
R8  10k  [0402-RES]  22.1,44.96 270 top
R9  10K, DNP  [0402-RES]  10.92,42.16 270 top
R10  4.7k  [0402-RES]  26.92,24.46 0 top
R11  4.7k  [0402-RES]  26.92,23.29 180 top
R12  4.7k  [0402-RES]  37.59,7.16 180 bottom
R13  4.7k  [0402-RES]  34.54,7.16 180 bottom
R14  4.7k  [0402-RES]  58.72,14.6 270 bottom
R15  33  [0402-RES]  38.61,35.86 0 bottom
R16  100K  [0402-RES]  63.88,37.85 0 bottom
R17  100K  [0402-RES]  63.88,36.7 0 bottom
R18  1M  [0402-RES]  36.58,24.51 90 top
R19  47k  [0402-RES]  67.94,9.78 0 bottom
R20  1M  [0402-RES]  36.58,29.59 90 top
R21  240  [0402-RES]  24.59,2.79 270 top
R22  240  [0402-RES]  23.55,2.79 270 top
R23  1.5K  [0402-RES]  23.67,20.83 90 bottom
R24  4.7k  [0402-RES]  13.41,43.56 180 bottom
R25  4.7k  [0402-RES]  67.94,10.92 180 bottom
R26  10K  [0402-RES]  3.28,14.86 270 bottom
R27  150  [0402-RES]  31.24,47.37 0 bottom
R28  150  [0402-RES]  27.18,46.74 90 bottom
R29  240  [0402-RES]  33.02,48.26 90 top
R30  240  [0402-RES]  42.04,44.2 270 bottom
R31  240  [0402-RES]  34.54,48.26 90 top
R32  240  [0402-RES]  29.84,48.26 90 top
R33  240  [0402-RES]  31.37,48.26 90 top
R34  150  [0402-RES]  27.18,44.45 270 bottom
R35  10K  [0402-RES]  4.32,14.86 270 bottom
R36  4.7k  [0402-RES]  67.06,27.56 0 top
R37  4.7k  [0402-RES]  67.06,29.84 0 top
R38  4.7k  [0402-RES]  67.06,32.13 0 top
R39  4.7k  [0402-RES]  67.06,34.42 0 top
R40  4.7k  [0402-RES]  67.06,36.7 0 top
R41  4.7k  [0402-RES]  67.06,38.99 0 top
R42  4.7k  [0402-RES]  67.06,41.27 0 top
R43  4.7k  [0402-RES]  67.06,43.56 0 top
R44  1k  [0402-RES]  40.89,44.2 270 bottom
R45  47k  [0402-RES]  54.84,48.72 180 bottom
R46  1K  [0402-RES]  53.77,50.42 270 bottom
R47  100k  [0402-RES]  55.42,46.53 180 bottom
R48  10k  [0402-RES]  55.85,51.56 90 bottom
R49  65k  [0402-RES]  56.9,51.56 270 bottom
R50  4.7k  [0402-RES]  67.06,26.42 0 top
R51  4.7k  [0402-RES]  67.06,28.7 0 top
R52  4.7k  [0402-RES]  67.06,30.99 0 top
R53  4.7k  [0402-RES]  67.06,33.27 0 top
R54  10K  [0402-RES]  9.55,34.14 90 bottom
R55  10K  [0402-RES]  7.9,33.71 180 bottom
R56  10K  [0402-RES]  2.24,14.86 270 bottom
R57  10K  [0402-RES]  7.9,34.75 180 bottom
R58  1.5K  [0402-RES]  20.29,21.54 180 bottom
R59  4.7k  [0402-RES]  50.39,10.77 180 bottom
R60  10K  [0402-RES]  22.3,15.67 180 bottom
R61  1K  [0402-RES]  25.63,2.79 90 top
R62  1K  [0402-RES]  26.67,2.79 90 top
R63  1K  [0402-RES]  27.71,2.79 90 top
R64  1K  [0402-RES]  28.75,2.79 90 top
R65  10K  [0402-RES]  15.88,17.27 270 bottom
R66  10K  [0402-RES]  38.61,34.72 180 bottom
R67  10K  [0402-RES]  28.57,40.51 90 top
R68  10K  [0402-RES]  34.29,40.51 90 top
R69  10K  [0402-RES]  33.15,40.51 90 top
R70  10K  [0402-RES]  32,40.51 90 top
R71  10K  [0402-RES]  36.58,40.51 90 top
R72  10K  [0402-RES]  37.72,40.51 90 top
R73  10K  [0402-RES]  35.43,40.51 90 top
R74  10K  [0402-RES]  30.86,40.51 90 top
R75  10K  [0402-RES]  29.72,40.51 90 top
R76  33  [0402-RES]  39.62,29.57 180 bottom
R77  33  [0402-RES]  67.06,45.85 0 top
R78  33  [0402-RES]  17.91,39.88 270 top
R79  33  [0402-RES]  19.3,39.88 270 top
R80  33  [0402-RES]  16.51,39.88 270 top
R81  33  [0402-RES]  15.11,39.88 270 top
R82  33  [0402-RES]  13.72,39.88 270 top
R83  33  [0402-RES]  12.32,39.88 270 top
R84  33  [0402-RES]  10.92,39.88 270 top
R85  33  [0402-RES]  19.38,25.78 180 top
R86  33  [0402-RES]  19.38,26.82 180 top
R87  100K  [0402-RES]  12.57,20.45 270 top
R88  100K  [0402-RES]  13.61,20.45 270 top
R89  1K, DNP  [0402-RES]  23.39,27.74 0 bottom
R90  1K  [0402-RES]  7.75,20.07 180 top
R91  240  [0402-RES]  21.34,23.77 180 top
R92  33  [0402-RES]  19.38,27.86 180 top
R93  33  [0402-RES]  23.24,36.45 180 top
R94  10K  [0402-RES]  38.61,33.58 180 bottom
R95  100K  [0402-RES]  21.21,6.73 180 bottom
R96  33  [0402-RES]  19.38,28.91 180 top
R97  33  [0402-RES]  19.38,29.95 180 top
R98  10K  [0402-RES]  16.51,42.16 270 top
R99  10K  [0402-RES]  15.11,42.16 270 top
R100  33  [0402-RES]  19.38,30.99 180 top
R101  10K  [0402-RES]  13.72,42.16 270 top
R102  10K  [0402-RES]  12.32,42.16 270 top
R103  10K  [0402-RES]  17.91,42.16 270 top
R104  120, DNP  [0603-RES]  41.81,11.91 90 bottom
R105  10K  [0402-RES]  19.3,42.16 270 top
R106  1.5K  [0402-RES]  23.24,37.59 180 top
R107  .1, 0805  [R0805]  16.15,45.09 90 bottom
R108  1K, DNP  [0402-RES]  23.39,28.88 0 bottom
R109  4.7k  [0402-RES]  57.56,14.6 90 bottom
R110  4.7k  [0402-RES]  56.39,14.6 270 bottom
R111  0  [0402-RES]  56.52,17.53 0 bottom
R112  0  [0603-RES]  7.62,36.93 0 bottom
R113  100K  [0402-RES]  63.88,29.84 0 bottom
R115  100K  [0402-RES]  63.88,30.99 0 bottom
R116  100K  [0402-RES]  67.06,44.7 0 top
R118  100K  [0402-RES]  63.88,28.7 180 bottom
R119  0, DNP  [0603-RES]  22.58,12.95 180 bottom
R120  100K  [0402-RES]  67.06,40.13 0 top
R121  0, DNP  [0603-RES]  17.91,10.34 270 bottom
R122  100K  [0402-RES]  67.06,42.42 0 top
R123  33  [0402-RES]  19.38,32.03 180 top
R124  33  [0402-RES]  19.38,33.07 180 top
R125  100K  [0402-RES]  67.06,35.56 180 top
R127  100K  [0402-RES]  67.06,37.85 180 top
R129  100K  [0402-RES]  63.88,35.56 0 bottom
R131  100K  [0402-RES]  63.88,32.13 0 bottom
R135  100K  [0402-RES]  63.88,34.42 0 bottom
R140  100K  [0402-RES]  63.88,33.27 180 bottom
R143  100K  [0402-RES]  56.03,41.71 90 bottom
R149  0  [0402-RES]  8.15,41.63 180 top
R150  0  [0402-RES]  38.61,32.51 0 bottom
R156  33  [0402-RES]  19.33,13.06 270 bottom
R158  10K  [0402-RES]  59.05,19.18 90 bottom
RST  SWITCH-MOMENTARY-2SMD-1101NE  [TACTILE-SWITCH-1101NE]  22.48,15.24 270 top
S1.1  JST_SH_6  [JST_SH_6]  53.34,4.57 0 top
S1.2  JST_SH_6  [JST_SH_6]  53.34,8.89 0 top
SD  SWITCH-MOMENTARY-2SMD-1101NE  [TACTILE-SWITCH-1101NE]  71.98,51.82 180 top
SIP  OSD3358  [BEAGLEBONE_BLUE_OSD3358]  51.82,28.96 90 top
TCK  TPSQB1,27  [B1,27]  48.64,13.46 0 bottom
TDI  TPSQB1,27  [B1,27]  50.42,13.46 0 bottom
TDO  TPSQB1,27  [B1,27]  49.53,11.94 0 bottom
TMS  TPSQB1,27  [B1,27]  51.31,11.94 0 bottom
TP1  TPSQB1,27  [B1,27]  58.93,42.06 180 bottom
TP5  TPB0,65  [BEAGLEBONE_BLUE_B0,65]  49.5,22.28 0 bottom
TP12  TPSQB1,27  [B1,27]  70.51,2.64 0 bottom
TRSTN  TPSQB1,27  [B1,27]  52.2,13.46 0 bottom
U1  TCAN1051HV  [BEAGLEBONE_BLUE_D8]  37.24,11.68 180 bottom
U2  SN74LV1T126DBVR  [BEAGLEBONE_BLUE_SOT23-5]  23.34,40.59 0 top
U3  TPD4S012DRY  [SON-6(TI)-DRY]  8.03,40.34 0 top
U4  TPD4S012DRY  [SON-6(TI)-DRY]  3.94,9.02 90 bottom
U5  24LC_32AT-I/OT  [SOT95P290X145-5N]  20.94,19.63 0 bottom
U6  SN74LVC1G07_DCK_5  [BEAGLEBONE_BLUE_DCK5]  37.21,12.75 0 top
U7  WL1835MODGBMOCT  [MOC-100(TI)]  11.33,30.86 180 top
U8  TPS2105_DBV_5  [DBV5]  20.7,9.91 90 bottom
U9  TXS0108ERGYR  [R-PVQFN-N20(TI)]  21.84,35.56 90 bottom
U10  TXS0108ERGYR  [R-PVQFN-N20(TI)]  23.24,29.24 270 top
U13  EMMC  [MICRON_EMMC_153]  31.62,34.44 0 bottom
U$2  [BATTERY_INDICATOR_LEFT]  32.26,45.21 0 top
U$5  [XYZ_BIG]  32.23,31.29 90 top
UT0  JST_SH_4  [JST_SH_4_SMD]  66.42,3.3 0 top
UT1  JST_SH_4  [JST_SH_4_SMD]  66.42,7.62 0 top
UT5  JST_SH_4  [JST_SH_4_SMD]  74.55,7.62 0 top
WIFI  GREEN  [BEAGLEBONE_BLUE_LED-0603]  22.83,22.73 90 top
WP  GHI2_TESTPAD/W_HOLE_1X1  [GHI2_TESTPAD/W_HOLE_1X1]  25.02,17.14 0 bottom
X2  SCHA5B0200  [SCHA5B0200]  1.4,25.02 90 bottom
X3  USB1  [USB_HOST_HORIZONTAL_W/CHASSIS_GND]  -2.54,9.02 270 top
X4  10118192-0001LF  [10118192-0001LF(MICRO-USB-B-AMPHENOL-FCI)]  1.45,38.35 90 bottom
Y1  24 MHz  [CRYSTAL_5X3.2MM]  34.16,29.59 90 top
Y2  32.768kHz  [CRYSTAL_3.2X1.5]  34.54,24.51 90 top

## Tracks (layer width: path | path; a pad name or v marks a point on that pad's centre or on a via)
3.3V  (via drill 0.25 pad 0.46, 0.5, 0.81 pad 0.41)
  Top 0.152: R10.1 v25.65,24.46 | C37.1 68.1,19.58 v68.76,19.58 | IMU.22 27.28,27.11 26.87,26.7 26.87,25.7 26.72,25.55 C8.1 | IMU.1 28.21,25.39 v27.96,25.15 | IMU.8 31.11,26.7 31.24,26.57 31.24,25.81 30.91,25.48 v30.91,25.15 | IMU.13 30.21,29.2 30.07,29.34 29.92,29.34 29.77,29.49 C9.2 | IMU.13 30.23,28.83 | IMU.13 31.77,28.8 32.54,28.04 32.54,26.01 v32.79,25.76 | R11.2 25.35,23.29 24.38,24.26 v24.38,24.89
  Top 0.254: CAN.2 45.18,12.43 45.52,12.09 v46.13,12.09 | 52.45,13.32 PWR.3 52.44,12.28 v52.78,11.94 | U10.19 v24.97,31.57 | C35.2 22.58,25.86 v22.2,25.48 | C56.1 v21.18,24.82 | v28.07,42.29 27.43,41.66 C39.1 R67.2 R75.2 R74.2 R70.2 R69.2 R68.2 R73.2 R71.2 R72.2 37.72,41.73 37.34,42.11 v36.73,42.11 | R122.2 68.25,42.42 68.56,42.72 v68.56,42.98 68.56,42.77 | R116.2 68.1,44.7 68.48,45.09 v68.48,45.87 | R120.2 68.12,40.13 68.5,40.51 v68.5,40.79 | S1.1.2 57.35,4.59 57.33,4.61 v57.33,7.7 57.33,8.88 S1.2.2 | v47.17,7.7 v47.18,7.71 GP0.2 | C13.1 30.96,24.43 30.75,24.65 BMP.8 30.41,24.2 v30.63,23.98 | C8.1 v25.45,25.55 | BMP.6 29.11,24.12 v29.26,23.98 29.26,23.88 29.76,23.37 BMP.2 | E3.2 E4.2 v83.11,42.39 | GP1.2 37.05,4.6 37.03,4.62 v37.03,6.15 37.03,8.87 I2C.2 | E2.2 v80.24,35.41 81.91,35.41 E1.2 | UT5.2 v74.02,6.98 | UT1.2 v65.89,7.7 | UT0.2 v65.89,5.77
  Top 0.406: C38.1 44.35,45.99 v44.35,44.83 | H1.20 v70.61,14.16 v70.61,14.17 | 15.24,21.77 v15.24,20.32 | H2.20 80.61,28.95 80.24,28.57 v79.78,28.57
  Bottom 0.152: R56.2 v2.23,13.54 | R26.2 v3.28,13.54 | U13.J10 30.85,33.69 v31.09,33.93 30.87,33.72 U13.K9 | U13.F5 32.37,35.19 | 32.37,35.19 U13.E6 32.61,35.93 v32.61,36.2 32.61,36.45 U13.C6 | 32.37,35.19 v32.16,34.98 | U13.P5 U13.N4 | U13.P3 U13.N4 | U13.N4 U13.M4 33.37,32.9 v33.35,32.92 | R140.2 v65.15,33.27 | R118.2 v65.15,28.7 | R109.1 57.56,14.45 57.71,14.6 v58.14,14.6 | v59.44,20.45 59.66,20.22 59.66,19.76 59.82,19.61 C41.1 | C27.1 v32.21,8.05 | C40.1 v48.9,8.43
  Bottom 0.254: C2.2 v76.2,21.01 | X2.4 2.66,16.89 v2.16,16.38 | R35.2 v4.32,13.54 | R65.2 v15.88,16 | R23.2 23.57,21.49 v22.45,21.49 | R58.2 20.9,21.49 v21.69,21.49 | 8.51,34.7 R54.2 10.19,34.7 10.46,34.42 10.46,33.2 10.29,33.02 9.93,33.02 8.13,31.22 8.13,29.82 6.86,28.55 6.86,22.45 8.81,20.5 9.75,20.5 13.59,24.33 18.47,24.33 v18.8,24.66 | R57.2 R55.2 | C34.2 v10.92,16.38 | C51.2 23.93,30.53 v24.97,31.57 | R66.2 R94.2 39.17,33.17 39.04,33.05 36.98,33.05 v36.8,33.22 | C49.2 38.91,38.86 38.73,38.68 v38.73,37.85 | C16.1 51.59,7.2 v51.59,8.2 | U9.19 24.26,33.81 v24.41,33.66 | U5.4 19.63,18.71 v19.63,19.38 | C28.1 19.86,17.7 v19.18,17.7 | R2.2 23.7,17.86 24.08,17.86 24.46,18.24 v24.46,18.52 | R60.2 23.32,15.67 v23.67,15.32 | U1.5 41.02,13.59 v41.2,13.77 | R13.1 v33.98,7.98 | R12.2 38.15,7.67 38.46,7.98 v38.84,7.98
  Bottom 0.305: 8.51,34.7 R57.2
  pour Route2 (rank 6): -2.54,57.15 88.9,57.15 88.9,-2.54 -2.54,-2.54
  pour Top: 38.86,36.58 40.13,36.58 40.39,36.83 40.39,37.21 39.75,37.21 39.75,38.48 40.39,38.48 40.39,38.86 40.13,39.12 38.86,39.12 37.97,38.23 37.97,37.47
  pour Top (no thermals): 14.61,24.89 15.75,24.89 15.75,21.08 14.61,21.08
5.0V  (via drill 0.25 pad 0.46, 0.5, 0.6)
  Top 0.254: GPS.5 v44.17,3 | PWR.4 51.44,9.09 50.7,8.36 v50.7,3
  Top 0.406: 5VREG.3 50.29,47.62 49.25,47.62 46.91,49.96 46.91,51.97 46.35,52.53 v46.35,53.42
  Route2 0.61: v77.09,9.88 78.16,10.95 78.16,15.49 79.38,16.71 80.47,16.71 81.56,17.8 81.56,32.97 82.5,33.91 83.59,33.91 v83.62,33.93
  Bottom 0.152: 46.35,51.9 47.12,51.9 L1.2 | U8.5 U8.1 21.65,6.85 R95.2
  Bottom 0.406: 46.35,51.9 v46.35,53.42
  Bottom 0.61: v77.09,9.88 75.92,8.71 72.9,8.71 67.18,3 v50.7,3 v44.17,3 23.67,3 22.55,4.12 22.55,10.41 C63.1 | v58.12,43.33 65.81,43.33 66.55,44.07 66.55,46.2 68.56,48.21 75.64,48.21 83.8,40.06 83.8,34.11 v83.62,33.93
  pour Top (isolate 0.152, no thermals): 57.02,40.64 59.31,40.64 59.31,43.94 52.83,43.94 52.83,45.59 50.8,45.59 50.8,47.75 49.78,47.75 49.78,45.03 52.07,45.03 52.07,43.43 57.02,43.43
  pour Bottom (rank 2, no thermals): 22.73,13.72 24.13,13.72 24.13,10.16 21.08,10.16 21.08,11.94 22.73,11.94
32.768KHZ
  Top 0.254: U7.36 7.83,24.08 7.52,23.77 7.26,23.77 7.07,23.58 OSC1.3
AIN0
  Top 0.152: SIP.B6 58.32,17.37 58.32,16.66 58.67,16.31 59.59,16.31 61.37,14.53 61.65,14.53 61.92,14.25 62.48,14.25 62.69,14.04 ADC.3
AIN1
  Top 0.152: SIP.C7 56.44,19.25 56.44,18.97 57.05,18.36 57.05,17.93 57.33,17.65 57.53,17.65 58.01,17.17 58.01,16.51 58.52,16 59.46,16 61.24,14.22 61.52,14.22 61.69,14.05 ADC.4
AIN2
  Top 0.152: ADC.5 60.69,14.34 59.33,15.7 57.05,15.7 56.74,16 56.74,17.17 56.26,17.65 SIP.B7
AIN3
  Top 0.152: SIP.A7 56.26,15.82 56.69,15.39 59.21,15.39 59.79,14.81 59.79,14.33 59.69,14.22 ADC.6
ALT.BUFF.OE  (via drill 0.25 pad 0.46)
  Top 0.152: v22.66,40.31 22.39,40.05 U2.1 22.39,38.41 22.68,38.12 R106.2 R93.2 22.68,34.67 22.38,34.37 22.38,32.72 22.61,32.49 v22.94,32.49 | U10.10 22.38,26.9 v21.74,26.9
  Bottom 0.152: U9.10 21.09,38.75 v22.66,40.31 | v21.74,26.9 21.74,30.33 22.43,31.01 22.43,31.98 v22.94,32.49
ANT1_A
  Top 0.406: U7.32 4.62,25.96 arc90 3.94,25.27 C48.2
ANT1_B
  Top 0.406: ANT1.SIG C48.1
ANT2_A
  Top 0.406: U7.18 4.62,35.76 arc-90 3.94,36.45 C58.2
ANT2_B
  Top 0.406: ANT2.SIG C58.1
BATT_LED_1  (via drill 0.25 pad 0.46)
  Top 0.152: B0.A 34.54,43.94 34.67,43.81 41.02,43.81 42.34,45.14 v42.72,45.14 | 50.32,36.37 v50.55,36.37 50.22,36.37 49.91,36.68 SIP.U12
  Bottom 0.152: v42.72,45.14 43.16,45.14 43.41,44.88 43.41,44.42 43.94,43.89 47.3,43.89 47.83,44.42 49.81,44.42 50.37,44.98 52.68,44.98 53.8,43.87 55.42,43.87 56.84,42.44 56.84,41.33 58.85,39.32 58.85,38.1 56.24,35.48 51.74,35.48 50.85,36.37 v50.55,36.37
BATT_LED_2  (via drill 0.25 pad 0.46)
  Top 0.152: B1.A 33.02,43.94 33.45,43.51 41.4,43.51 42.37,44.48 v42.72,44.48 | SIP.T5 58.32,36.42 58.32,39.06 v58.37,39.12
  Bottom 0.152: 58.37,39.24 v58.37,39.12 | 58.37,39.09 v58.37,39.12 | v58.37,39.12 58.37,39.32 56.54,41.15 56.54,41.55 56.39,41.71 56.16,41.71 56.03,41.83 R143.2 56.03,42.77 55.24,43.56 53.67,43.56 52.55,44.68 50.49,44.68 49.94,44.12 47.95,44.12 47.42,43.59 43.81,43.59 42.93,44.48 v42.72,44.48
BATT_LED_3  (via drill 0.25 pad 0.46)
  Top 0.152: B2.A 31.37,43.89 32.05,43.2 41.76,43.2 42.37,43.81 v42.72,43.81 | SIP.V6 57.53,38.94 v57.71,39.12
  Bottom 0.152: v57.71,39.12 57.71,39.24 57,39.95 56.03,39.95 55.55,40.44 55.55,42.49 54.79,43.26 53.54,43.26 52.43,44.37 50.62,44.37 50.06,43.81 48.08,43.81 47.55,43.28 43.69,43.28 43.16,43.81 v42.72,43.81
BATT_LED_4  (via drill 0.25 pad 0.46)
  Top 0.152: B3.A 29.84,43.89 30.84,42.9 42.47,42.9 v42.72,43.16 | SIP.T11 51.18,36.52 50.67,37.03 v50.55,37.03
  Bottom 0.152: v42.72,43.16 42.9,42.98 47.7,42.98 48.23,43.51 50.19,43.51 50.75,44.07 52.3,44.07 53.42,42.95 54.66,42.95 55.24,42.37 55.24,40.31 55.91,39.65 56.64,39.65 57.05,39.24 57.05,38.84 57.38,38.51 57.38,37.08 56.08,35.79 51.92,35.79 50.67,37.03 v50.55,37.03
BATT_MID
  Bottom 0.406: R44.1 R30.1 42.04,47.47 LIPO.P$2 38.94,47.37 R27.1
BATT_MINUS
  Bottom 0.254: BAL.6 BAL.5 | C1.2 C18.1 30.84,41.66 BAL.5 | PROT.6 34.07,43.09 | 34.07,43.09 35.01,44.03 PROT.2 35.01,45.12 34.8,45.34 34.67,45.34 34.42,45.59 Q1.3 | BAL.5 31.88,42.8 32.26,43.18 C19.2 33.27,43.89 34.07,43.09 | 37.09,46.1 37.08,46.09 Q1.1
  Bottom 0.406: C15.1 39.75,45.64 LIPO.P$3 38.94,46.43 38.61,46.1 37.09,46.1 | Q1.3 Q1.2 Q1.1
BT_AUD_CLK
  Top 0.152: U10.1 22.49,31.99 22.4,32.08 20.8,32.08 20.52,32.36 20.52,32.92 20.37,33.07 R124.1
BT_AUD_FSYNC
  Top 0.152: R123.1 20.37,32.03 20.78,31.62 20.78,30.68 20.98,30.48 U10.3
BT_AUD_IN
  Top 0.152: R97.1 20.37,29.95 20.83,29.48 U10.5
BT_AUD_OUT
  Top 0.152: R100.1 20.32,30.99 20.47,30.84 20.47,30.3 20.79,29.98 U10.4
BT_EN  (via drill 0.25 pad 0.46)
  Top 0.152: SIP.K17 43.03,28.32 42.82,28.52 v42.82,28.96 | v26.72,35.31 25.93,35.31 24.94,34.31 v24.46,34.31
  Route2 0.152: v42.82,28.96 42.32,29.46 40.49,29.46 39.14,30.81 31.67,30.81 29.26,33.22 29.26,34.87 28.85,35.28 26.75,35.28 v26.72,35.31
  Bottom 0.152: v24.46,34.31 v24.45,34.31 U9.18
BT_EN_1V8  (via drill 0.25 pad 0.46)
  Top 0.152: v11.94,25.35 11.66,25.35 11.33,25.02 U7.41 11.33,24.11 11.48,23.95 11.96,23.95 13.61,22.3 R88.1
  Bottom 0.152: v11.94,25.35 11.94,26.09 12.19,26.34 16.64,26.34 17.32,27.03 17.32,34.09 18.09,34.85 18.87,34.85 19.41,34.31 U9.3
BT_HCI_CTS
  Top 0.152: R86.1 20.37,26.82 20.5,26.95 20.5,27.56 20.92,27.98 U10.8
BT_HCI_RTS
  Top 0.152: R85.1 20.34,25.78 20.8,26.24 20.8,27.3 20.98,27.48 U10.9
BT_HCI_RX
  Top 0.152: R96.1 20.02,28.98 U10.6
BT_HCI_TX
  Top 0.152: R92.1 20.32,27.86 20.94,28.48 U10.7
CANH  (via drill 0.25 pad 0.46)
  Top 0.152: v44.15,12.14 44.15,13.3 CAN.3
  Bottom 0.152: v44.15,12.14 43.07,11.06 R104.1 39.71,11.06 U1.7
CANL  (via drill 0.25 pad 0.46)
  Top 0.152: v43.2,12.14 43.2,13.31 CAN.4
  Bottom 0.152: v43.2,12.14 42.58,12.76 R104.2 41.24,12.76 40.79,12.32 U1.6
CGND
  Bottom 0.305: X2.CGND5 14.19,27.59 13.21,28.57 13.21,31.62 12.56,32.27 11.84,32.27 | 11.84,32.27 X2.CGND4 11.15,32.32 11.24,32.32 11.3,32.26 | X3.5 9.92,17.77 X2.CGND1 12.4,19.89 14.1,21.59 X2.CGND6 | 4.01,35.25 X4.CGND6 4.04,35.3 4.04,35.31 11.73,35.31 12.01,35.03 12.01,33.1 11.81,32.89 11.81,32.34 11.86,32.29 11.84,32.27
  pour Bottom (rank 6): -3.81,58.42 -3.81,26.67 1.65,26.67 1.65,30.86 2.03,31.24 2.03,32.89 2.79,33.78 4.7,33.78 4.7,36.2 2.92,36.2 2.92,40.51 4.7,40.51 4.7,42.55 2.54,44.7 2.54,51.05 4.45,52.96 11.18,52.96 11.81,52.32 11.81,49.66 14.86,46.99 14.86,45.34 17.4,45.34 17.4,47.12 16.51,47.12 16.51,48.89 17.4,50.04 17.4,53.34 74.68,52.96 76.45,51.18 76.45,48.01 79.38,45.09 82.42,45.09 84.71,42.8 84.71,26.67 90.17,26.67 90.17,58.42
  pour Bottom (rank 6): -3.81,26.67 -3.81,-3.81 90.17,-3.81 90.17,26.67 84.71,26.67 84.71,22.48 82.55,20.32 82.55,12.45 76.83,6.73 76.83,3.3 75.18,1.65 19.18,1.65 17.91,2.92 17.91,4.19 16.26,5.84 13.34,5.84 11.18,3.68 9.78,3.68 7.37,6.1 3.05,6.1 2.41,6.73 2.41,11.05 3.3,11.94 6.99,11.94 9.65,14.6 9.65,16.38 8.64,17.4 6.6,17.4 5.08,15.62 5.08,13.21 4.83,12.95 1.91,12.95 1.65,13.21 1.65,16.76 2.03,17.14 2.03,18.41 1.65,18.8 1.65,26.67
  pour Top (rank 6): -3.81,58.42 -3.81,26.67 1.65,26.67 1.65,49.78 4.83,52.96 11.68,52.96 12.32,52.32 12.32,49.78 13.34,48.77 15.88,48.77 17.27,50.16 17.27,52.96 73.91,52.96 77.47,49.4 77.47,47.37 79.5,45.34 84.33,45.34 84.96,44.7 84.96,26.67 90.17,26.67 90.17,58.42
  pour Top (rank 6): -3.81,26.67 -3.81,-3.81 90.17,-3.81 90.17,26.67 84.96,26.67 85.09,11.94 82.8,9.02 79.5,9.02 77.85,7.37 77.85,4.7 74.8,1.65 17.4,1.65 17.4,4.19 16,5.97 13.34,5.97 11.68,4.32 9.53,4.32 6.6,7.24 6.6,11.81 9.78,14.99 9.78,16.26 8.51,17.53 1.65,17.53 1.65,26.67
CHG_EN
  Top 0.152: 22.12,45.54 R8.1
  Top 0.254: CHGIC.6 22.12,45.54 | R8.1 R7.2
CO  (via drill 0.25 pad 0.46)
  Top 0.254: R7.1 27.61,44.4 v28.07,43.94
  Bottom 0.254: v28.07,43.94 28.07,43.05 28.32,42.8 BAL.8
DCAN1_RX  (via drill 0.25 pad 0.46)
  Top 0.152: 45.06,14.91 v45.06,14.53 45.06,15.11 45.44,15.49 45.44,16.41 45.31,16.53 45.31,19.76 45.16,19.91 44.78,19.91 44.35,20.34 44.35,21.56 43.94,21.97 SIP.E17 | v41,8.69 38.73,10.95 v37.47,10.95
  Bottom 0.152: v45.06,14.53 45.59,13.99 45.59,7.44 45.06,6.91 44.12,6.91 43.54,7.49 43.54,8.33 43,8.87 41.17,8.87 v41,8.69 | v37.47,10.95 36.52,11.89 36.52,13.26 36.2,13.59 U1.4
DCAN1_SILENT  (via drill 0.25 pad 0.46)
  Top 0.152: SIP.M16 45.34,30.86 45.82,30.38 47.3,30.38 48.16,29.52 48.16,29.39 48.44,29.11 48.62,29.11 49.43,28.3 49.43,26.95 48.74,26.26 48.44,26.26 48.16,25.98 48.16,24.23 48.36,24.03 48.67,24.03 v49.28,23.42 | v39.73,16.2 39.73,15.57 v38.25,14.1
  Bottom 0.152: v49.28,23.42 49.28,22.96 48.74,22.43 45.9,22.43 45.34,21.87 45.34,18.59 45.62,18.31 46.97,18.31 47.4,17.88 47.4,16.89 46.99,16.48 46.53,16.48 45.82,17.2 40.72,17.2 v39.73,16.2 | v38.25,14.1 38.25,10.03 38.51,9.78 U1.8
DCAN1_TX  (via drill 0.25 pad 0.46)
  Top 0.152: v43.08,14.53 43.08,21.18 SIP.E18
  Bottom 0.152: v43.08,14.53 43.08,14.25 44.68,12.65 44.68,9.73 44.12,9.17 37.16,9.17 36.55,9.78 U1.1
DO
  Bottom 0.254: PROT.1 34.04,44.7 33.53,44.7 33.15,45.09 Q1.4
EMMC_RST  (via drill 0.25 pad 0.46)
  Top 0.152: SIP.R14 46.63,33.93 46.63,33.05 46.35,32.77 v45.92,32.77
  Bottom 0.152: U13.K5 33.39,33.71 37.39,33.71 37.52,33.58 R94.1 38.48,33.58 38.61,33.71 38.61,35.05 38.84,35.28 39.47,35.28 41.1,36.91 42.72,36.91 43.87,35.76 44.2,35.76 44.78,35.18 45.19,35.18 45.31,35.05 45.31,34.44 45.74,34.01 45.74,32.94 v45.92,32.77
EQEP_0A  (via drill 0.25 pad 0.46)
  Top 0.152: v56.9,22.15 57.2,22.45 66.04,22.45 66.75,23.16 66.75,24.66 68.02,25.93 68.68,25.93 69.34,26.59 v69.34,27.28 | SIP.B12 49.43,18.64 49.43,20.95 49.66,21.18 51.44,21.18 51.66,20.95 51.66,20.34 52.09,19.91 52.65,19.91 52.96,19.61 v53.09,19.61 | v79.45,34.06 79.79,34.4 E1.3
  Bottom 0.152: v56.9,22.15 56.57,21.82 54.59,21.82 54.33,21.56 54.33,20.5 54.43,20.4 54.43,19.81 54.1,19.48 53.21,19.48 v53.09,19.61 | v69.34,27.28 69.52,27.46 70.61,27.46 70.87,27.71 70.87,29.23 71.63,30 72.67,30 73.25,30.58 73.25,31.9 73.86,32.51 75.69,32.51 77.24,34.06 v79.45,34.06
EQEP_0B  (via drill 0.25 pad 0.46)
  Top 0.152: v66.42,25.07 66.42,23.29 65.89,22.76 56.82,22.76 v56.77,22.81 | v53.9,20.07 53.49,20.07 53.34,20.22 52.25,20.22 51.97,20.5 51.97,21.18 51.66,21.49 49.48,21.49 49.12,21.13 49.12,19.91 SIP.C13 | v79.45,33.4 E1.4
  Bottom 0.152: v66.42,25.07 66.42,25.86 66.9,26.34 69.09,26.34 69.9,27.15 70.74,27.15 71.22,27.63 71.22,29.06 71.86,29.69 72.8,29.69 73.56,30.45 73.56,31.77 73.99,32.21 75.87,32.21 77.06,33.4 v79.45,33.4 | v56.77,22.81 56.08,22.12 54.46,22.12 54.03,21.69 54.03,20.19 v53.9,20.07
EQEP_1A  (via drill 0.25 pad 0.46)
  Top 0.152: SIP.V2 63.02,38.48 v63.25,38.71 | E2.3 77,34.4 76.78,34.62 76.78,38.73 75.64,39.88 v74.78,39.88
  Bottom 0.152: v63.25,38.71 63.25,37.92 R16.2 63.8,37.85 63.88,37.92 63.88,38.23 64.16,38.51 66.57,38.51 67.67,39.6 74.5,39.6 v74.78,39.88
EQEP_1B  (via drill 0.25 pad 0.46)
  Top 0.152: SIP.V3 61.65,38.18 v62.03,38.18 | E2.4 76.94,33.4 76.48,33.86 76.48,36.4 75.82,37.06 74.5,37.06 v74.02,37.54
  Bottom 0.152: v62.03,38.18 62.38,38.18 62.79,37.77 62.79,37.47 62.99,37.26 63.17,37.26 63.32,37.11 R17.2 63.68,36.7 63.88,36.91 63.88,37.08 64.06,37.26 66.27,37.26 66.37,37.36 73.84,37.36 v74.02,37.54
EQEP_2A  (via drill 0.25 pad 0.46)
  Top 0.152: SIP.T12 50.32,35.94 v50.55,35.71 | E3.3 77.83,41.4 76.71,41.4 76.53,41.58 76.53,44.48 75.87,45.14 73.97,45.14 v73.79,45.31
  Bottom 0.152: v50.55,35.71 50.9,35.71 51.44,35.18 56.36,35.18 59.99,38.81 59.99,40.36 60.96,41.33 65.73,41.33 67.84,43.43 67.84,44.48 68.5,45.14 73.61,45.14 v73.79,45.31
EQEP_2B  (via drill 0.25 pad 0.46)
  Top 0.152: SIP.R12 50.34,34.67 50.55,34.87 v50.55,35.05 | E3.4 76.76,40.39 76.05,41.1 76.05,44.22 75.49,44.78 73.99,44.78 v73.81,44.6
  Bottom 0.152: v50.55,35.05 51.1,35.05 51.28,34.87 56.49,34.87 60.3,38.68 60.3,40.23 61.09,41.02 65.86,41.02 68.15,43.31 68.15,44.3 68.63,44.78 73.64,44.78 v73.81,44.6
GND  (via drill 0.25 pad 0.46, 0.41, 0.5)
  Top 0.152: U10.11 | C37.2 68.54,20.71 v68.76,20.5 | IMU.20 27.32,27.91 27.18,27.76 27.18,27.43 26.95,27.2 26.54,27.2 26.39,27.05 C8.2 | IMU.9 31.19,27.11 31.34,26.95 31.6,26.95 31.73,26.82 C6.2 31.73,25.68 31.62,25.58 v31.62,25.15 | IMU.18 28.21,29.2 28.35,29.34 28.5,29.34 28.65,29.49 C9.1 | IMU.18 28.18,28.83 | v27.76,29.39 27.76,29.03 27.99,28.8 IMU.18
  Top 0.254: H2.3 | H2.4 | H2.10 83.84,22.52 | PWR.1 54.44,12.27 v54.1,11.94 | PWR.2 v53.44,11.94 | CAN.1 46.13,13.28 46.13,14.27 v45.87,14.53 | R6.1 20.95,46.23 v20.45,46.74 | CHGIC.8 23.75,47.07 v24,46.81 | C10.1 25.45,52.53 v25.15,52.83 | R32.2 R33.2 R29.2 R31.2 35.13,48.82 35.43,48.51 v35.43,47.98 | 5VREG.8 v47.75,53.42 | 5VREG.7 v49.02,53.42 | 5VREG.6 v50.29,53.42 | 5VREG.5 v51.56,53.39 | R127.1 v68.33,37.85 | R52.2 v68.33,30.99 | R51.2 v68.33,28.7 | R53.2 v68.33,33.27 | U10.11 v23.44,27 | R8.2 22.1,43.94 22.35,43.69 v26.16,43.69 | U2.3 v24.28,40.39 | R106.1 23.8,37.92 v24.13,38.25 | C50.2 23.37,33.4 23.57,33.2 23.57,32.18 v23.24,31.85 | U10.TP v23.24,31.17 | C35.1 23.99,25.97 U10.11 | R125.1 68.05,35.56 68.33,35.84 v68.33,36.07 | v48.18,7.7 GP0.1 | GPS.2 47.17,4.58 v47.17,6.76 | S1.1.1 v58.34,7.7 S1.2.1 | R50.2 68.17,26.42 v68.58,26.82 | SIP.A18 42.29,15.14 v41.68,14.53 | GPS.6 43.18,5.87 v42.9,6.15 | BMP.1 30.7,23.05 30.96,23.32 C13.2 31.7,23.32 32.03,23.65 v32.03,23.98 | C8.2 25.78,26.67 v25.45,26.34 | BMP.5 28.46,24.93 28.73,25.2 29.52,25.2 29.76,24.95 BMP.7 29.76,24.26 29.92,24.11 v29.92,23.98 | C36.2 36.04,34.04 35.89,33.88 v35.89,33.22 | C39.2 v27.43,39.09 | C4.1 17.6,44.4 v17.48,44.27 | 6VREG.3 55.82,46.5 55.65,46.33 55.65,45.8 55.5,45.64 v55.5,45.49 | C7.2 16.02,44.93 v17.45,44.93 | 14.09,45.34 C12.2 13.55,45.07 v13.28,45.34 | C56.2 23.47,24.82 v23.82,24.46 | E3.1 E4.1 v83.11,43.38 | SD.1 75.13,50.39 v75.77,49.76 | E2.1 v80.24,36.4 E1.1 | GP1.1 38.05,4.6 38,4.66 v38,6.15 38,8.84 I2C.1 | UT5.1 v75.01,6.96 | SIP.V1 63.88,38.99 63.12,39.75 SIP.W2 | UT1.1 v66.88,7.7 | UT0.1 v66.88,5.77 | ADC.1 65.46,13.21 v65.71,12.95 | SIP.A1 64.19,17.2 v64.19,17.48
  Top 0.254: POW.1 v17.4,16.81 | MOD.1 v26.34,18.39 | v26.34,18.39 | RST.1 21.84,19.02 v20.7,19.02 | U6.3 36.19,12.12 v37.21,12.12 | PAU.1 31.6,18.39 31.37,18.16 v31.37,16 | H2.9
